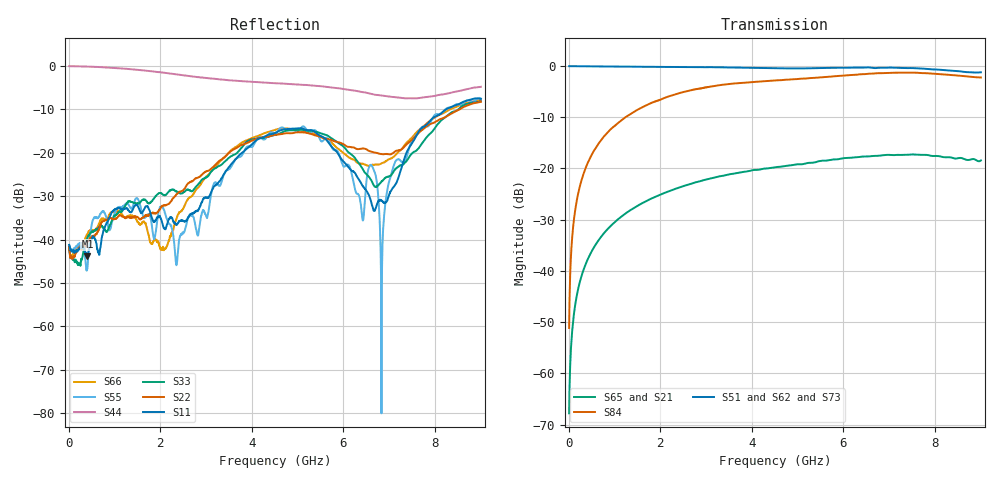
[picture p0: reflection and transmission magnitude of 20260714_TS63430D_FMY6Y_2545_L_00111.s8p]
# GHz S DB R 50
! CMT, SN0916, 25263762, 26.7.0
! Date: 15.07.2026 14:55:18
! Data: Format
! Freq S1.1:dB/Ang S1.2:dB/Ang S1.3:dB/Ang S1.4:dB/Ang S1.5:dB/Ang S1.6:dB/Ang S1.7:dB/Ang S1.8:dB/Ang
!  S2.1:dB/Ang S2.2:dB/Ang S2.3:dB/Ang S2.4:dB/Ang S2.5:dB/Ang S2.6:dB/Ang S2.7:dB/Ang S2.8:dB/Ang
!  S3.1:dB/Ang S3.2:dB/Ang S3.3:dB/Ang S3.4:dB/Ang S3.5:dB/Ang S3.6:dB/Ang S3.7:dB/Ang S3.8:dB/Ang
!  S4.1:dB/Ang S4.2:dB/Ang S4.3:dB/Ang S4.4:dB/Ang S4.5:dB/Ang S4.6:dB/Ang S4.7:dB/Ang S4.8:dB/Ang
!  S5.1:dB/Ang S5.2:dB/Ang S5.3:dB/Ang S5.4:dB/Ang S5.5:dB/Ang S5.6:dB/Ang S5.7:dB/Ang S5.8:dB/Ang
!  S6.1:dB/Ang S6.2:dB/Ang S6.3:dB/Ang S6.4:dB/Ang S6.5:dB/Ang S6.6:dB/Ang S6.7:dB/Ang S6.8:dB/Ang
!  S7.1:dB/Ang S7.2:dB/Ang S7.3:dB/Ang S7.4:dB/Ang S7.5:dB/Ang S7.6:dB/Ang S7.7:dB/Ang S7.8:dB/Ang
!  S8.1:dB/Ang S8.2:dB/Ang S8.3:dB/Ang S8.4:dB/Ang S8.5:dB/Ang S8.6:dB/Ang S8.7:dB/Ang S8.8:dB/Ang
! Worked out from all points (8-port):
!   2001 points, 10 MHz to 9 GHz, reference 50 ohm
!   strongest paths, dB at 10 MHz, 2.257 GHz, 4.505 GHz, 6.753 GHz, 9 GHz:
!     S51: -0.1, -0.2, -0.5, -0.4, -1.3
!     S62: -0.1, -0.3, -0.5, -0.4, -1.2
!     S73: -0.1, -0.3, -0.5, -0.5, -1.2
!     S84: -51.1, -5.8, -2.9, -1.5, -2.3
!     S65: -67.8, -24.2, -19.8, -17.6, -18.5
!     S21: -67.5, -24.2, -19.8, -17.5, -18.4
!   lowest |S11| = -43.9 dB at 410.1 MHz (marker M1), VSWR 1.01, Z = 50.3 - j0.581 ohm
!   |S11| at or under -10 dB: start of sweep to 8.236 GHz
